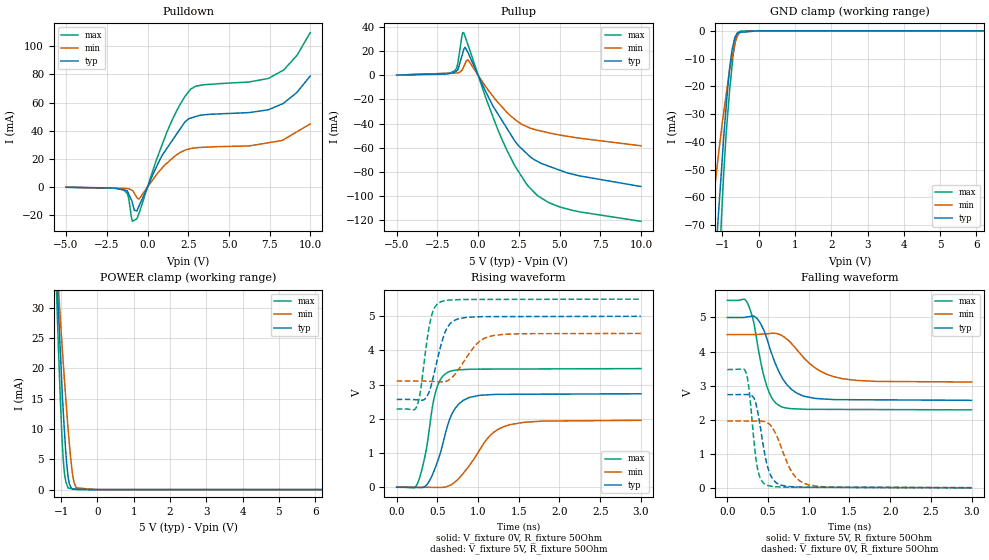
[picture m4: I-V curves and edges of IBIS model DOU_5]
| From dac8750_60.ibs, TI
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[Model] DOU_5  |5V digital 3-state output
Model_type   3-state
Polarity   Non-Inverting
Vmeas = 2.5
Vref = 2.5
Cref = 0pF
Rref = 50
|   typ   min   max
|   (nom PVT)   (Fast PVT)   (slow PVT)
|   BUFFER OUTPUT TURNED HIGH
C_comp   1.746E-12   1.362E-12   2.109E-12
|   BUFFER OUTPUT LOW
|C_comp   1.630E-12   1.294E-12   1.996E-12
|   BUFFER HIGH Z STATE
|C_comp   1.507E-12   1.318E-12   1.528E-12
| Where   nom PVT is  Nominal Process, 5.0V, 36C
|   Fast PVT is Strong Process, 5.5V, -40C
|   Slow PVT is Weak Process, 4.5V, 134C
|C_comp - from L-C Tank method, L = 1nH, peak frequency
[Voltage Range]   5   4.5   5.5
|Operating Temperature   27   125   -40
|Junction Temperature
[Temperature Range]   36   134   -40
[Pullup Reference]   5   4.5   5.5
[Pulldown Reference]   0   0   0
[Power Clamp Reference]   5   4.5   5.5
[GND Clamp Reference]   -0   0   0
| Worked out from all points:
|   slope of the pulldown table from 0 to 0.75 V, typ, clamps not added: 39.2 ohm
|   slope of the pullup table from 0 to 0.75 V, typ, clamps not added: 35.3 ohm
|   GND clamp passes 1 mA (typ) near -0.60 V on its own axis
|   POWER clamp passes 1 mA (typ) near -0.77 V on its own axis
|   falling waveform, V_fixture 5V, R_fixture 50Ohm: 20-80 % time 256ps typ, 382ps min, 169ps max; typ from 5 V to 2.57 V
|   rising waveform, V_fixture 0V, R_fixture 50Ohm: 20-80 % time 218ps typ, 359ps min, 149ps max; typ from 0.005 V to 2.73 V
|   rising waveform, V_fixture 5V, R_fixture 50Ohm: 20-80 % time 159ps typ, 254ps min, 114ps max; typ from 2.57 V to 5 V
|   falling waveform, V_fixture 0V, R_fixture 50Ohm: 20-80 % time 126ps typ, 213ps min, 89.2ps max; typ from 2.73 V to 0.005 V
[Pulldown]
|   Voltage   I(typ)   I(min)   I(max)
-5V       -197.5uA   -139.9uA   -199.2uA
-1.449V   -2.145mA   -1.036mA   -2.111mA
-1.154V   -5.012mA   -1.315mA   -8.127mA
-930.9mV  -11.28mA   -2.486mA   -24.39mA
-663.8mV  -17.05mA   -7.261mA   -22.69mA
-504.4mV  -13.08mA   -8.346mA   -18.17mA
1.189V    27.48mA    16.95mA    39.01mA
2.641V    48.94mA    27.27mA    69.48mA
7.419V    54.89mA    31.45mA    77.12mA
8.373V    59.76mA    33.82mA    83.36mA
9.182V    67.46mA    39.34mA    93.72mA
9.985V    78.88mA    44.83mA    109.7mA
[GND Clamp]
|   Voltage   I(typ)   I(min)   I(max)
-5V       -964.1mA   -649.3mA   -1.343A
-1.457V   -136.7mA   -87.39mA   -199.1mA
-1.249V   -93.02mA   -61.01mA   -133.7mA
-1.121V   -68.5mA    -46.03mA   -94.86mA
-1.113V   -66.95mA   -45.09mA   -92.54mA
-1.026V   -50.35mA   -35.64mA   -67.68mA
-909.8mV  -29.48mA   -24.34mA   -39.71mA
-802.7mV  -13.77mA   -14.31mA   -21.82mA
-734.3mV  -6.894mA   -9.856mA   -12.67mA
-637.8mV  -1.914mA   -3.8mA     -3.147mA
-506.2mV  -543.6uA   -450.3uA   -111.9uA
9.985V    0A         0A         0A
[Pullup]
|   Voltage   I(typ)   I(min)   I(max)
-5V       264.4uA    209.5uA    285.1uA
-1.401V   3.043mA    1.903mA    4.234mA
-1.239V   4.862mA    2mA        10.55mA
-987.5mV  16.49mA    4.326mA    33.31mA
-883.9mV  21.59mA    7.332mA    35.27mA
-601.2mV  18.2mA     12.55mA    24.44mA
1.328V    -34.49mA   -24.14mA   -48.97mA
2.288V    -55.23mA   -36.83mA   -75.89mA
3.114V    -66.54mA   -43.31mA   -92.59mA
4.277V    -75.05mA   -47.51mA   -105.2mA
5.112V    -79.18mA   -49.71mA   -109.6mA
9.985V    -92.19mA   -58.41mA   -121mA
[POWER Clamp]
|   Voltage   I(typ)   I(min)   I(max)
-5V       613.9mA    474.2mA    818.2mA
-1.154V   40.05mA    41.31mA    37.77mA
-1.113V   34.65mA    37.04mA    30.35mA
-1.081V   30.55mA    33.98mA    24.7mA
-1.026V   23.42mA    28.66mA    15.69mA
-979.1mV  17.34mA    24.4mA     9.083mA
-939.4mV  12.81mA    20.86mA    4.856mA
-898.8mV  8.83mA     17.38mA    2.311mA
-803.4mV  1.972mA    9.73mA     241.3uA
-682.6mV  110uA      2.461mA    143.3uA
-583.5mV  29.46uA    279.7uA    62.78uA
9.985V    0A         0A         0A
[Ramp]
R_load = 50
|   typ   min   max
dV/dt_r   1.63726/2.17058e-010   1.17071/3.57596e-010   2.08122/1.48946e-010
dV/dt_f   1.45746/2.55165e-010  0.834968/3.79914e-010   1.92655/1.68438e-010
[Falling Waveform]
V_fixture = 5V
V_fixture_min = 4.5V
V_fixture_max = 5.5V
R_fixture = 50Ohm
C_fixture = 0F
|   Time   V(typ)   V(min)   V(max)
0s        4.998V     4.498V     5.5V
246.1ps   5.015V     4.499V     5.426V
322.4ps   5.037V     4.499V     4.878V
362.4ps   4.976V     4.499V     4.331V
481.4ps   4.407V     4.522V     3.011V
559.6ps   3.84V      4.537V     2.59V
655.3ps   3.311V     4.486V     2.39V
852.2ps   2.781V     4.058V     2.317V
1.303ns   2.591V     3.265V     2.302V
3ns       2.569V     3.106V     2.289V
[Rising Waveform]
V_fixture = 0V
V_fixture_min = 0V
V_fixture_max = 0V
R_fixture = 50Ohm
C_fixture = 0F
|   Time   V(typ)   V(min)   V(max)
0s        5.292mV    7.466mV    1.254mV
255.8ps   -5.275mV   3.048mV    112mV
362ps     59.2mV     1.213mV    1.08V
477.5ps   595.7mV    -782.5uV   2.784V
627.1ps   1.82V      31.87mV    3.362V
717.8ps   2.306V     160.4mV    3.423V
818.7ps   2.542V     411.8mV    3.441V
1.107ns   2.702V     1.408V     3.455V
1.311ns   2.718V     1.769V     3.457V
3ns       2.734V     1.959V     3.47V
[Rising Waveform]
V_fixture = 5V
V_fixture_min = 4.5V
V_fixture_max = 5.5V
R_fixture = 50Ohm
C_fixture = 0F
|   Time   V(typ)   V(min)   V(max)
0s        2.569V     3.105V     2.289V
249.1ps   2.557V     3.105V     2.375V
293.3ps   2.548V     3.104V     2.831V
420ps     2.944V     3.097V     4.937V
539.5ps   4.117V     3.084V     5.419V
600.5ps   4.569V     3.095V     5.46V
698.1ps   4.864V     3.257V     5.479V
988.1ps   4.982V     4.203V     5.49V
1.183ns   4.989V     4.433V     5.491V
3ns       4.998V     4.497V     5.5V
[Falling Waveform]
|Gnd
V_fixture = 0V
V_fixture_min = 0V
V_fixture_max = 0V
R_fixture = 50Ohm
C_fixture = 0F
|   Time   V(typ)   V(min)   V(max)
0s        2.734V     1.959V     3.47V
229.5ps   2.738V     1.962V     3.382V
269.3ps   2.734V     1.963V     2.84V
325.5ps   2.64V      1.964V     1.421V
366.4ps   2.306V     1.964V     623.9mV
475.7ps   805.7mV    1.927V     84.79mV
600.5ps   148.5mV    1.558V     32.66mV
798.6ps   34.14mV    438mV      18.61mV
994.8ps   20.66mV    89.56mV    17.06mV
3ns       5.297mV    7.64mV     1.254mV
